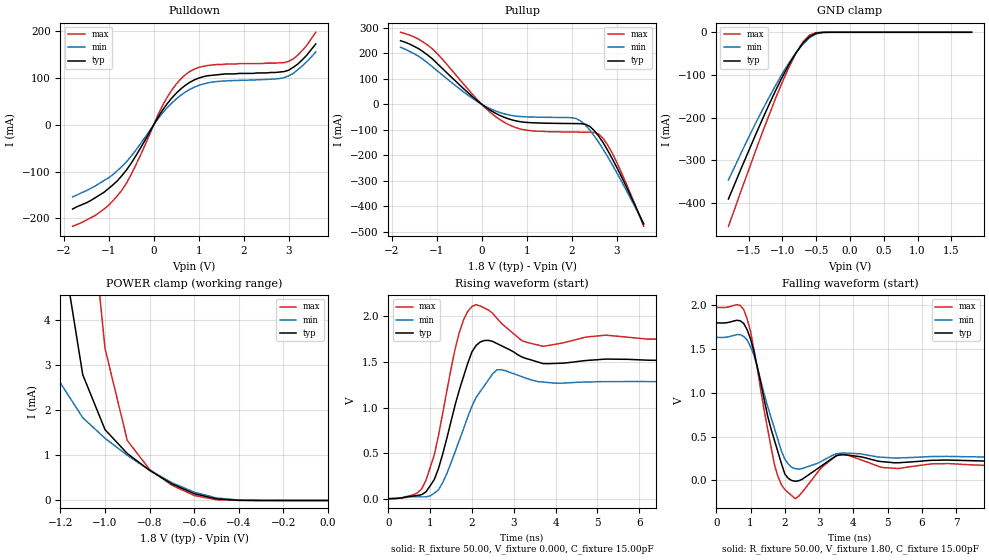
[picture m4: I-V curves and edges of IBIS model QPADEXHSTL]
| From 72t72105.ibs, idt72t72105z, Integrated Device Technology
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|   Model QPADEXHSTL
[Model]   QPADEXHSTL
Model_type   3-state
Polarity   Non-Inverting
Enable   Active-High
Vmeas =  0.900V
C_comp   3.00pF   NA   NA
[Temperature Range]   25.00   85.00   -40.00
[Voltage Range]   1.80V   1.60V   2.00V
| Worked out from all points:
|   slope of the pulldown table from 0 to 0.27 V, typ, clamps not added: 6.57 ohm
|   slope of the pullup table from 0 to 0.27 V, typ, clamps not added: 8.55 ohm
|   GND clamp passes 1 mA (typ) near -0.45 V on its own axis
|   POWER clamp passes 1 mA (typ) near -0.89 V on its own axis
|   rising waveform, R_fixture 50.00, V_fixture 0.000, C_fixture 15.00pF: 20-80 % time 537ps typ, 631ps min, 486ps max; typ from 0 V to 1.52 V
|   falling waveform, R_fixture 50.00, V_fixture 1.80, C_fixture 15.00pF: 20-80 % time 547ps typ, 590ps min, 481ps max; typ from 1.8 V to 0.223 V
[Pulldown]
| voltage   I(typ)   I(min)   I(max)
-1.8V     -180mA     -154mA     -217mA
-1.1V     -144mA     -119mA     -180mA
-700mV    -108mA     -88.57mA   -139mA
-400mV    -66.98mA   -54.66mA   -86.64mA
200mV     31.71mA    25.58mA    41.77mA
400mV     57.04mA    46.47mA    74.01mA
700mV     84.35mA    69.78mA    107mA
1.2V      105mA      89.75mA    127mA
2.7V      112mA      98.23mA    132mA
3V        117mA      105mA      136mA
3.3V      139mA      126mA      159mA
3.6V      173mA      156mA      198mA
[Pullup]
| voltage   I(typ)   I(min)   I(max)
-1.8V     249mA      223mA      282mA
-1.1V     179mA      148mA      218mA
-100mV    14.11mA    10.85mA    18.81mA
500mV     -51.24mA   -37.65mA   -70.6mA
1V        -71.51mA   -49.75mA   -102mA
2V        -75.96mA   -53.01mA   -109mA
2.2V      -76.47mA   -65.69mA   -110mA
2.4V      -86.66mA   -101mA     -110mA
2.6V      -125mA     -149mA     -117mA
2.8V      -181mA     -206mA     -160mA
3.1V      -282mA     -300mA     -266mA
3.6V      -470mA     -469mA     -479mA
[GND_clamp]
| voltage   I(typ)   I(min)   I(max)
-1.8V     -391mA     -346mA     -455mA
-1.5V     -278mA     -246mA     -323mA
-1.3V     -205mA     -183mA     -236mA
-1.1V     -136mA     -124mA     -154mA
-1V       -104mA     -96.2mA    -116mA
-900mV    -74.56mA   -70.77mA   -80.61mA
-800mV    -48.24mA   -47.87mA   -49.04mA
-700mV    -26.16mA   -28.23mA   -23.28mA
-600mV    -10.07mA   -12.98mA   -6.406mA
-500mV    -2.002mA   -3.724mA   -655uA
-400mV    -177uA     -538uA     -28.11uA
1.8V      18.12nA    77.44nA    18nA
[POWER_clamp]
| voltage   I(typ)   I(min)   I(max)
-1.8V     60.33mA    37.96mA    93.88mA
-1.3V     11.23mA    4.427mA    25.79mA
-1.2V     5.851mA    2.598mA    15.98mA
-1.1V     2.782mA    1.831mA    8.297mA
-1V       1.566mA    1.375mA    3.362mA
-900mV    1.038mA    999uA      1.326mA
-800mV    666uA      671uA      687uA
-700mV    367uA      394uA      337uA
-600mV    151uA      184uA      111uA
-500mV    35.57uA    56.06uA    16.17uA
-400mV    4.038uA    9.226uA    1.082uA
0V        18.12nA    21.07nA    20nA
[Ramp]
| variable   typ   min   max
dV/dt_r   0.92/0.43n   0.78/0.56n   1.07/0.36n
dV/dt_f   0.96/0.43n   0.83/0.48n   1.10/0.35n
R_load = 50.00
[Rising Waveform]
R_fixture = 50.00
V_fixture = 0.000
C_fixture = 15.00pF
R_dut = 0.75
L_dut = 8.10nH
C_dut = 0.53pF
| time   V(typ)   V(min)   V(max)
0s        0V         0V         0V
700ps     34.88mV    21.64mV    65.11mV
900ps     75.3mV     20mV       201mV
1.2ns     332mV      97.2mV     694mV
1.7ns     1.196V     643mV      1.826V
2.1ns     1.681V     1.111V     2.128V
2.6ns     1.701V     1.414V     1.977V
3.7ns     1.482V     1.279V     1.672V
5.2ns     1.531V     1.284V     1.793V
9.9ns     1.52V      1.283V     1.759V
[Falling Waveform]
R_fixture = 50.00
V_fixture = 1.80
C_fixture = 15.00pF
R_dut = 0.75
L_dut = 8.10nH
C_dut = 0.53pF
| time   V(typ)   V(min)   V(max)
0s        1.8V       1.634V     1.977V
800ps     1.793V     1.644V     1.951V
1ns       1.615V     1.525V     1.699V
1.7ns     452mV      588mV      171mV
2ns       70.24mV    240mV      -107mV
2.3ns     -11.66mV   132mV      -211mV
3.1ns     173mV      224mV      156mV
3.6ns     289mV      309mV      300mV
5.3ns     200mV      254mV      134mV
9.9ns     223mV      268mV      177mV
